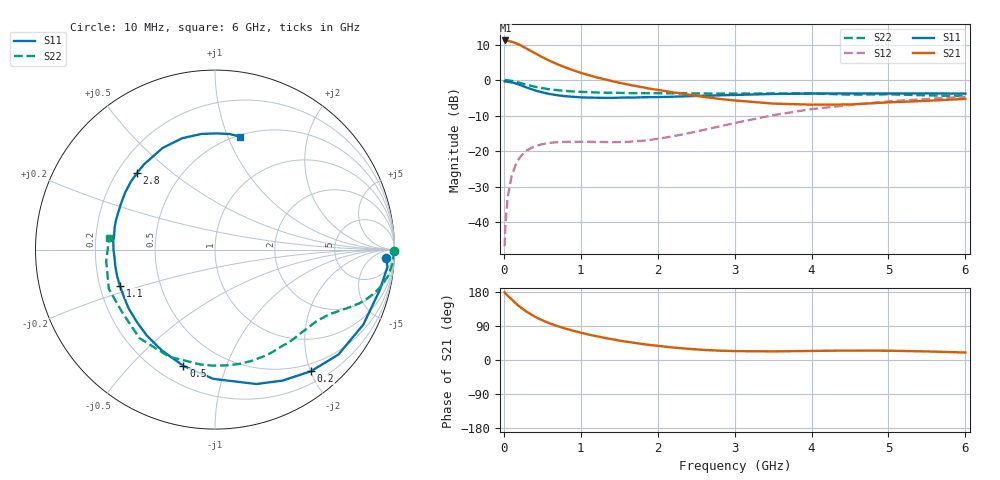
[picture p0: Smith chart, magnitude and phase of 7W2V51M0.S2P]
! Infineon Technologies  Discrete & RF Semiconductors
! BFS17W
! Si NPN RF Bipolar Junction Transistor in SOT323
! VCE = 2.5 V  IC = 1 mA
! Common Emitter S-Parameters:  August  1999
# GHz  S  MA  R  50
!  f  S11  S21  S12  S22
! GHz  MAG  ANG  MAG  ANG  MAG  ANG  MAG  ANG
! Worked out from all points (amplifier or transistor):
!   36 points, 10 MHz to 6 GHz, reference 50 ohm
!   highest |S21| = 11.2 dB at 20 MHz (marker M1)
!   |S21| within 3 dB of that: start of sweep to 355.8 MHz
!   unconditionally stable (mu >= 1): 1.015 GHz to end of sweep
!   at 250 MHz: K = 0.26, MSG = 15.1 dB, |S12| = -20.7 dB
!   at 1.4 GHz: K = 1.29, MAG = 5.4 dB, |S12| = -17.5 dB
!   at 6 GHz: K = 1.11, MAG = -2.3 dB, |S12| = -4.7 dB
!   S11 on the Smith chart (normalised r, x): 10 MHz: 21, -22; 200 MHz: 0.38, -2.00; 500 MHz: 0.30, -0.72; 1.1 GHz: 0.28, -0.17; 2.8 GHz: 0.28, +0.38; 6 GHz: 0.51, +1.11
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0.01  0.9563 -2.7  3.587 178.7  0.0046 90.7  0.9999 -0.4
0.02  0.9656 -5.8  3.611 176.0  0.009 85.0  0.9955 -1.7
0.05  0.9454 -13.8  3.568 169.7  0.0224 81.7  0.992 -4.4
0.1  0.9261 -26.8  3.465 160.2  0.0442 74.7  0.9763 -8.6
0.15  0.9027 -40.4  3.324 150.4  0.0629 66.8  0.9484 -12.3
0.2  0.8629 -51.8  3.158 141.8  0.0792 61.2  0.9192 -15.4
0.25  0.8213 -62.7  2.95 134.0  0.092 55.1  0.8873 -18.1
0.3  0.7835 -72.9  2.76 126.9  0.1028 50.4  0.8596 -20.3
0.4  0.7201 -90.8  2.406 114.6  0.1171 42.9  0.8072 -23.8
0.5  0.6713 -105.2  2.104 104.8  0.1255 37.5  0.77 -26.4
0.6  0.6351 -117.8  1.859 96.3  0.1311 34.1  0.7409 -28.7
0.8  0.593 -137.5  1.509 82.9  0.1353 30.2  0.7039 -33.3
1.1  0.5669 -159.3  1.177 67.2  0.1356 29.4  0.6758 -40.4
1.6  0.5689 175.2  0.871 48.1  0.1349 37.2  0.6563 -53.9
2.2  0.5835 153.7  0.673 32.9  0.162 52.3  0.6528 -71.9
2.8  0.6092 135.5  0.544 24.7  0.2224 60.0  0.6466 -91.0
3.5  0.6371 117.3  0.467 22.8  0.3206 58.4  0.6491 -113.2
4  0.6469 106.4  0.451 23.9  0.3903 52.9  0.6483 -130.5
4.5  0.6489 96.8  0.454 25.0  0.445 46.5  0.6241 -146.1
5  0.6474 89.4  0.486 24.5  0.5023 40.1  0.6305 -159.8
5.5  0.6492 82.8  0.511 22.7  0.5425 33.7  0.6096 -173.9
6  0.6451 77.5  0.544 19.7  0.5803 27.8  0.5934 174.0
